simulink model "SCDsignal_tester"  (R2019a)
settings: Solver=FixedStepDiscrete  StartTime=0.0  StopTime=10.0  RelTol=1e-3

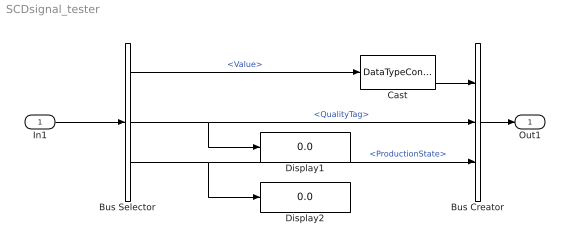
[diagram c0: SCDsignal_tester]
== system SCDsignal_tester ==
  In1 : Inport  OutDataTypeStr=Bus: SCDbusToBeTested  Interpolate=off
  Bus Creator : BusCreator  Inputs=3  OutDataTypeStr=Bus: SCDbusToBeTested
  Bus Selector : BusSelector  OutputSignals=Value,QualityTag,ProductionState
  Cast : DataTypeConversion
  Display1 : Display
  Display2 : Display
  Out1 : Outport  OutDataTypeStr=Bus: SCDbusToBeTested
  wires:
  In1/1 -> Bus Selector/1
  Bus Selector/1 -> Cast/1  "<Value>"
  Bus Selector/3 -> Bus Creator/3, Display2/1  "<ProductionState>"
  Bus Selector/2 -> Display1/1, Bus Creator/2  "<QualityTag>"
  Bus Creator/1 -> Out1/1
  Cast/1 -> Bus Creator/1
